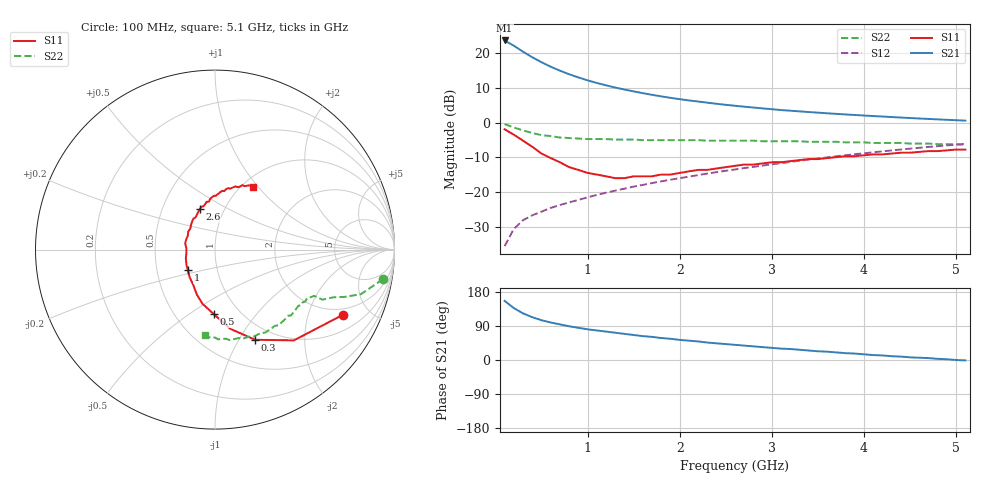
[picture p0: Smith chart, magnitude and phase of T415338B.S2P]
!AT-41533
!S and NOISE PARAMETERS at Vce=8V  Ic=5mA.  LAST UPDATED 01-25-95
# ghz s ma r 50
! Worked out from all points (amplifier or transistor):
!   51 points, 100 MHz to 5.1 GHz, reference 50 ohm
!   highest |S21| = 23.5 dB at 100 MHz (marker M1)
!   |S21| within 3 dB of that: start of sweep to 287.2 MHz
!   unconditionally stable (mu >= 1): 903.3 MHz to 2.394 GHz
!   at 900 MHz: K = 1.00, MSG = 17.5 dB, |S12| = -22.2 dB
!   at 2.6 GHz: K = 0.97, MSG = 9.1 dB, |S12| = -13.4 dB
!   at 5.1 GHz: K = 0.82, MSG = 3.3 dB, |S12| = -6.1 dB
!   lowest NFmin = 0.70 dB at 100 MHz
!   S11 on the Smith chart (normalised r, x): 100 MHz: 1.68, -3.39; 300 MHz: 0.82, -1.18; 500 MHz: 0.76, -0.63; 1 GHz: 0.72, -0.17; 2.6 GHz: 0.77, +0.36; 5.1 GHz: 1.12, +0.94
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0.1  0.8 -27.0  14.95 156.0  0.017 77.0  0.95 -10.0
0.2  0.67 -49.0  12.57 137.0  0.03 67.0  0.85 -17.0
0.3  0.55 -66.0  10.32 123.0  0.04 63.0  0.77 -20.0
0.4  0.45 -79.0  8.6 113.0  0.047 62.0  0.71 -22.0
0.5  0.36 -91.0  7.304 105.0  0.053 61.0  0.66 -25.0
0.6  0.31 -103.0  6.293 99.0  0.06 61.0  0.64 -25.0
0.7  0.27 -112.0  5.531 94.0  0.066 62.0  0.61 -25.0
0.8  0.23 -122.0  4.912 89.0  0.072 63.0  0.6 -26.0
0.9  0.21 -132.0  4.425 85.0  0.078 64.0  0.59 -27.0
1  0.19 -143.0  4.015 81.0  0.085 64.0  0.58 -28.0
1.1  0.18 -152.0  3.686 78.0  0.092 65.0  0.58 -29.0
1.3  0.16 -174.0  3.169 72.0  0.106 66.0  0.57 -31.0
1.4  0.16 177.0  2.967 69.0  0.113 66.0  0.57 -32.0
1.6  0.17 160.0  2.632 63.0  0.128 66.0  0.56 -34.0
1.8  0.18 146.0  2.368 58.0  0.144 66.0  0.56 -36.0
2  0.19 135.0  2.163 53.0  0.16 65.0  0.56 -38.0
2.3  0.21 121.0  1.923 46.0  0.186 64.0  0.55 -42.0
2.6  0.24 111.0  1.737 40.0  0.213 63.0  0.55 -47.0
3.1  0.27 97.0  1.509 30.0  0.262 59.0  0.54 -55.0
3.5  0.3 89.0  1.385 23.0  0.306 56.0  0.53 -63.0
4.3  0.36 74.0  1.198 10.0  0.399 47.0  0.51 -79.0
5.1  0.41 59.0  1.065 -1.0  0.495 37.0  0.48 -97.0
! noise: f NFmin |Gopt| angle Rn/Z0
0.1  0.7  0.6  7  0.19
0.9  1  0.34  80  0.13
1.8  1.4  0.35  -168  0.08
2.4  1.6  0.52  -127  0.15
